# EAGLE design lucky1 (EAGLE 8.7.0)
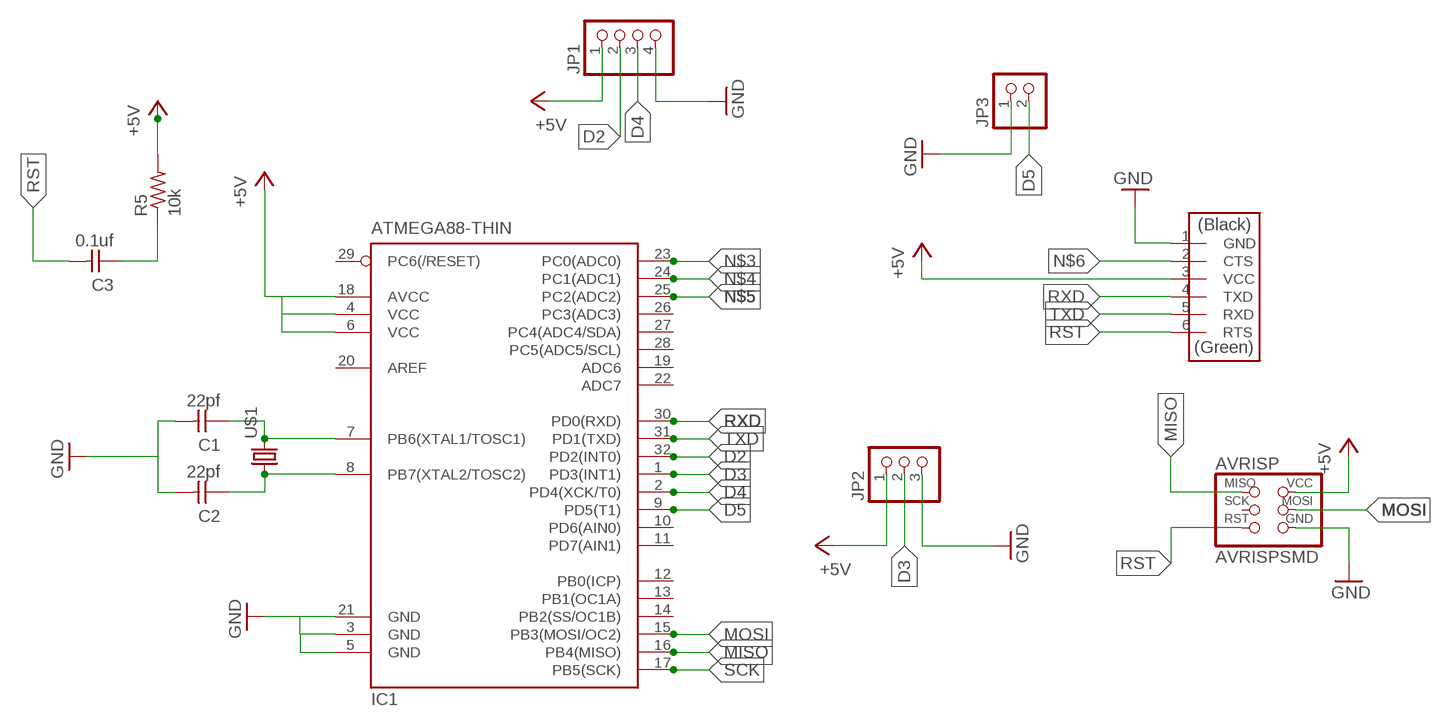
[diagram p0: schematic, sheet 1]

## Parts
AVRISP  AVRISPSMD  [2X03SMD]
C1  22pf  CAP-UNPOLARIZED  [C1206]
C2  22pf  CAP-UNPOLARIZED  [C1206]
C3  0.1uf  CAP-UNPOLARIZED  [C1206]
FTDI  FTDI-SMD-HEADER  [1X06SMD]
IC1  ATMEGA88-THIN  [TQFP32-08THIN]
JP1  PINHD-1X4  [1X04]
JP2  PINHD-1X3  [1X03]
JP3  PINHD-1X2  [1X02]
R5  10k  RES-US1206FAB  [R1206FAB]
U$1  CRYSTALHC49UP  [HC49UP]

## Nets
+5V: AVRISP.2(VCC) FTDI.3(VCC) IC1.4(VCC) IC1.6(VCC) IC1.18(AVCC) JP1.1 JP2.1 R5.2
D2: IC1.32(PD2(INT0)) JP1.2
D3: IC1.1(PD3(INT1)) JP2.2
D4: IC1.2(PD4(XCK/T0)) JP1.3
D5: IC1.9(PD5(T1)) JP3.2
GND: AVRISP.6(GND) C1.2 C2.2 FTDI.1(GND) IC1.3(GND) IC1.5(GND) IC1.21(GND) JP1.4 JP2.3 JP3.1
MISO: AVRISP.1(MISO) IC1.16(PB4(MISO))
MOSI: AVRISP.4(MOSI) IC1.15(PB3(MOSI/OC2))
N$1: C1.1 IC1.7(PB6(XTAL1/TOSC1)) U$1.2
N$2: C2.1 IC1.8(PB7(XTAL2/TOSC2)) U$1.1
N$3: IC1.23(PC0(ADC0))
N$4: IC1.24(PC1(ADC1))
N$5: IC1.25(PC2(ADC2))
N$6: FTDI.2(CTS)
N$8: C3.1 R5.1
RST: AVRISP.5(RST) C3.2 FTDI.6(RTS)
RXD: FTDI.4(TXD) IC1.30(PD0(RXD))
SCK: IC1.17(PB5(SCK))
TXD: FTDI.5(RXD) IC1.31(PD1(TXD))
Unconnected: AVRISP.3(SCK) IC1.10(PD6(AIN0)) IC1.11(PD7(AIN1)) IC1.12(PB0(ICP)) IC1.13(PB1(OC1A)) IC1.14(PB2(SS/OC1B)) IC1.19(ADC6) IC1.20(AREF) IC1.22(ADC7) IC1.26(PC3(ADC3)) IC1.27(PC4(ADC4/SDA)) IC1.28(PC5(ADC5/SCL)) IC1.29(PC6(/RESET))

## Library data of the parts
AVRISP = fab:AVRISP
C1-C3 = fab:CAP-UNPOLARIZED
FTDI = fab:FTDI-SMD-HEADER
IC1 = fab:ATMEGA88-THIN
JP1 = pinhead:PINHD-1X4: PIN HEADER
JP2 = pinhead:PINHD-1X3: PIN HEADER
JP3 = pinhead:PINHD-1X2: PIN HEADER
R5 = fab:RES-US: Resistor (US Symbol)
U$1 = crystal:CRYSTAL: CRYSTAL; OC_FARNELL: unknown; OC_NEWARK: unknown

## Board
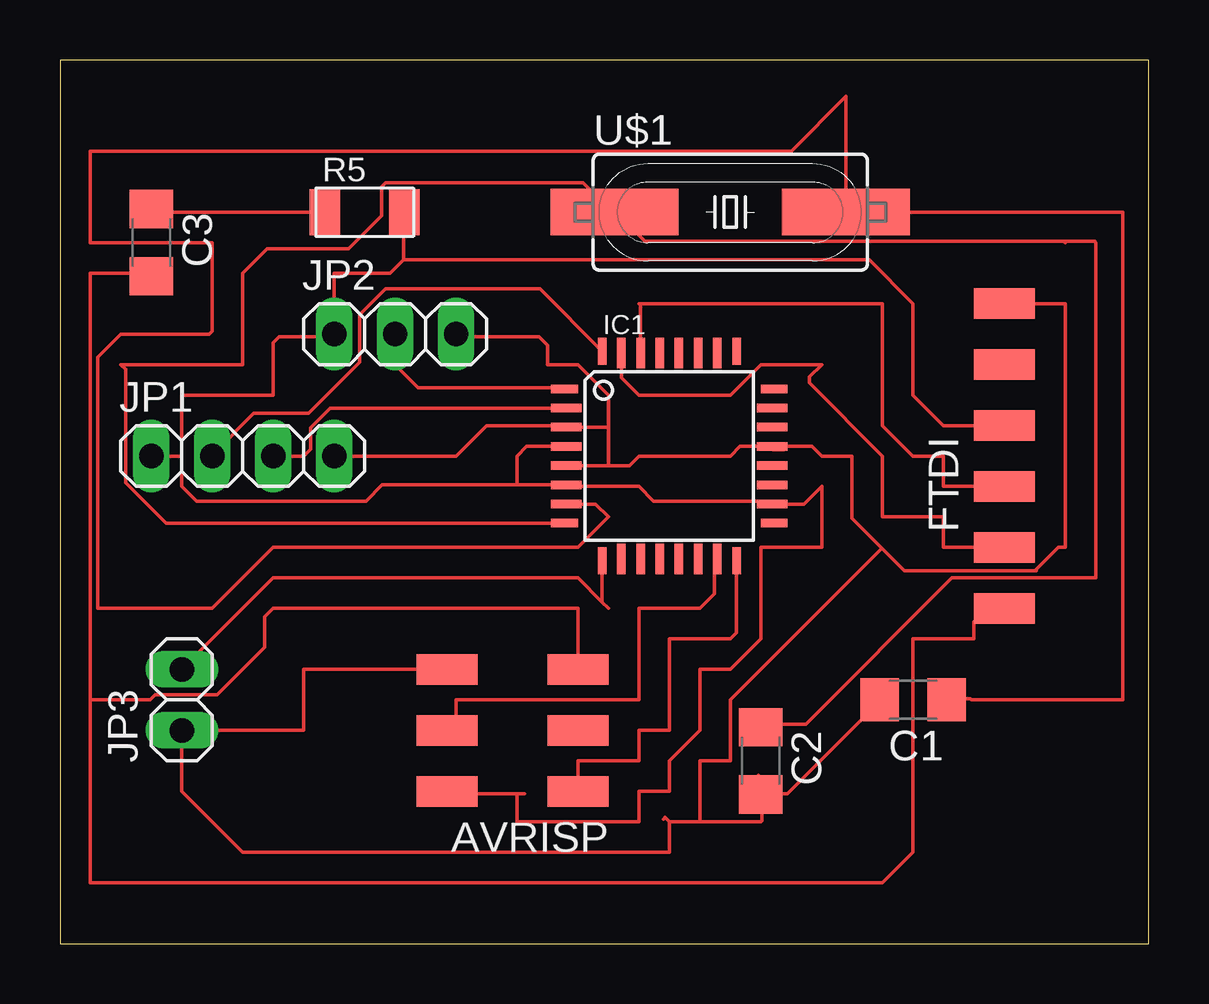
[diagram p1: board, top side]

Size 45.39 x 36.82 mm. Coordinates in mm from the lower left corner, seen from the top.
Outline: 0,0 45.39,0 45.39,36.82 0,36.82 0,0
Copper layers (1*16): Top 0.035mm / dielectric 1.5mm / Bottom 0.035mm
Design rules "default": minimum track width 6mil, minimum drill 0.35mm, track to track 6mil, track to pad 6mil, pad to pad 6mil, via to via 6mil, smd to smd 6mil, copper to edge 40mil, drill to drill 6mil, minimum pad ring 10mil, minimum via ring 8mil, stop-mask expansion 4mil, vias tented up to drill 0mil, thermal gap 10mil

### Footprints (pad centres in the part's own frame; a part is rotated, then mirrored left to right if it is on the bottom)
2X03SMD = smd 2.54 x 1.27: 1 -2.54,2.54; 2 2.92,2.54; 3 -2.54,0; 4 2.92,0; 5 -2.54,-2.54; 6 2.92,-2.54
C1206 = smd 1.6 x 1.8: 1 -1.4,0; 2 1.4,0
1X06SMD = smd 2.54 x 1.27: 1 0,6.35; 2 0,3.81; 3 0,1.27; 4 0,-1.27; 5 0,-3.81; 6 0,-6.35
TQFP32-08THIN = smd 1.118 x 0.356: 1 -4.369,2.8; 8 -4.369,-2.8; 17 4.369,-2.8; 24 4.369,2.8 | smd 1.27 x 0.356: 2 -4.293,2; 3 -4.293,1.2; 4 -4.293,0.4; 5 -4.293,-0.4; 6 -4.293,-1.2; 7 -4.293,-2; 18 4.293,-2; 19 4.293,-1.2; 20 4.293,-0.4; 21 4.293,0.4; 22 4.293,1.2; 23 4.293,2 | smd 0.356 x 1.118: 9 -2.8,-4.369; 16 2.8,-4.369; 25 2.8,4.369; 32 -2.8,4.369 | smd 0.356 x 1.27: 10 -2,-4.293; 14 1.2,-4.293; 15 2,-4.293; 26 2,4.293; 27 1.2,4.293; 31 -2,4.293 | smd 0.35 x 1.27: 11 -1.2,-4.293; 12 -0.4,-4.293; 13 0.4,-4.293; 28 0.4,4.293; 29 -0.4,4.293; 30 -1.2,4.293
1X04 = drill 1.016 long: 1 -3.81,0; 2 -1.27,0; 3 1.27,0; 4 3.81,0
1X03 = drill 1.016 long: 1 -2.54,0; 2 0,0; 3 2.54,0
1X02 = drill 1.016 long: 1 -1.27,0; 2 1.27,0
R1206FAB = smd 1.27 x 1.905: 1 -1.651,0; 2 1.651,0
HC49UP = smd 5.334 x 1.93: 1 -4.826,0; 2 4.826,0

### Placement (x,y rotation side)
AVRISP  19.05,8.89 180 top
C1  35.56,10.16 180 top
C2  29.21,7.62 270 top
C3  3.81,29.21 270 top
FTDI  39.37,20.32 0 top
IC1  25.4,20.32 0 top
JP1  7.62,20.32 0 top
JP2  13.97,25.4 0 top
JP3  5.08,10.16 90 top
R5  12.7,30.48 0 top
U$1  27.94,30.48 0 top

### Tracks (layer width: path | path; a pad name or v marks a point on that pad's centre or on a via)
+5V
  Top 0.152: 20.57,19.2 21.03,19.2 IC1.6 | IC1.6 21.18,19.05 24.13,19.05 24.74,18.44 29.57,18.44 IC1.18 31.02,18.32 31.75,19.05 31.75,16.51 29.21,16.51 29.21,12.7 27.94,11.43 26.67,11.43 26.67,8.89 25.4,7.62 25.4,6.35 24.13,6.35 24.13,5.08 19.05,5.08 19.05,6.25 | 19.36,6.25 19.05,6.25 | 19.05,6.25 16.15,6.25 AVRISP.2 | 14.33,28.5 14.33,30.48 R5.2 | JP2.1 11.43,25.6 | 39.32,21.64 FTDI.3 36.83,21.59 35.56,22.86 35.56,26.67 33.73,28.5 14.33,28.5 | 4.27,20.42 3.96,20.42 | 3.96,20.42 3.81,20.42 JP1.1 | JP2.1 11.43,25.3 9.14,25.3 8.89,25.04 8.89,22.86 5.08,22.86 5.08,20.32 | 3.96,20.42 JP1.1 | JP1.1 5.08,20.32 | 5.08,20.32 5.08,19.05 5.69,18.44 12.75,18.44 13.43,19.12 19.05,19.12 | 14.33,28.5 13.77,27.94 11.43,27.94 JP2.1 | 19.05,19.12 IC1.6 | 19.05,19.12 19.05,20.32 19.45,20.72 IC1.4
D2
  Top 0.152: JP1.2 6.4,20.42 8.08,22.1 10.36,22.1 12.5,24.23 12.5,26.21 13.56,27.28 17.78,27.28 18.44,27.28 20.01,27.28 IC1.32
D3
  Top 0.152: IC1.1 21.03,23.16 16.51,23.16 16.15,23.16 14.94,23.16 13.97,24.13 13.97,25.35 | JP2.2 13.97,25.35 | 13.97,25.35 14.02,25.3
D4
  Top 0.152: IC1.2 11.27,22.32 10.44,21.49 10.44,20.6 10.16,20.32 JP1.3
D5
  Top 0.152: 22.55,15.85 IC1.9 22.6,14.23 | 5.18,11.43 JP3.2 8.89,15.24 21.59,15.24 22.6,14.23 | 22.6,14.23 22.86,13.97
GND
  Top 0.152: 5.64,8.99 5.18,8.99 JP3.1 | 29.26,6.25 30.33,6.25 34.14,10.06 C1.2 | 29.26,6.25 C2.2 29.11,6.25 29.11,7.01 | 21.49,19.96 21.18,19.96 IC1.5 22.86,19.92 | 21.18,21.49 IC1.3 | 29.57,20.73 IC1.21 | 39.47,26.36 39.47,26.67 FTDI.1 41.91,26.67 41.91,16.51 41.6,16.51 40.64,15.54 | 40.64,15.54 35.2,15.54 34.27,16.48 | 40.64,15.54 40.69,15.54 | 30.18,20.57 29.72,20.57 IC1.21 | 11.43,20.42 JP1.4 16.51,20.32 17.78,21.59 20.93,21.59 21.03,21.49 IC1.3 | JP2.3 16.61,25.3 19.96,25.3 20.32,24.94 20.32,24.13 21.59,24.13 22.86,22.86 22.86,21.59 | 25.15,5.18 25.22,5.26 25.4,5.08 | IC1.21 28.34,20.72 27.94,20.32 24.13,20.32 23.73,19.92 22.86,19.92 | IC1.3 22.79,21.52 22.86,21.59 | 22.86,21.59 22.86,19.92 | 25.4,5.08 25.4,3.81 7.62,3.81 5.08,6.35 JP3.1 | 34.27,16.48 33.02,17.73 33.02,20.32 31.75,20.32 31.35,20.72 IC1.21 | 29.26,6.25 29.26,5.13 29.21,5.08 26.67,5.08 | 26.67,5.08 25.4,5.08 | 34.27,16.48 27.94,10.16 27.94,7.62 26.67,7.62 26.67,5.08 | JP3.1 10.16,8.89 10.16,11.43 AVRISP.6
MISO
  Top 0.152: IC1.16 28.19,15.85 28.19,12.95 27.94,12.7 25.4,12.7 25.4,8.89 24.13,8.89 24.13,7.62 21.59,7.62 AVRISP.1
MOSI
  Top 0.152: IC1.15 27.28,16 27.28,15.24 27.28,14.78 27.28,14.58 26.67,13.97 24.13,13.97 24.13,10.16 16.51,10.16 16.51,9.27 AVRISP.4 16.15,8.99
N$1
  Top 0.152: 21.18,18.29 IC1.7 22.32,18.32 22.86,17.78 21.59,16.51 8.89,16.51 6.35,13.97 1.57,13.97 1.57,24.43 2.54,25.4 6.22,25.4 6.35,25.53 6.35,29.21 1.27,29.21 1.27,33.02 30.48,33.02 32.77,35.31 U$1.2 44.3,30.48 44.3,10.16 38,10.16 37.95,10.21 37.03,10.21 C1.1
N$2
  Top 0.152: IC1.8 4.42,17.53 2.74,19.2 2.74,23.93 2.54,24.13 7.62,24.13 7.62,27.94 8.64,28.96 12.04,28.96 13.41,30.33 13.41,31.55 13.56,31.7 21.79,31.7 23.01,30.48 U$1.1 23.16,30.48 24.38,29.26 41.86,29.26 | C2.1 29.26,9.14 31.09,9.14 37.19,15.24 43.18,15.24 43.18,29.21 43.13,29.26 41.86,29.26 | 41.86,29.26 41.91,29.21
N$8
  Top 0.152: R5.1 3.81,30.48 C3.1
RST
  Top 0.152: 21.49,11.43 AVRISP.5 21.59,13.97 8.89,13.97 8.53,13.61 8.53,12.34 6.55,10.36 3.96,10.36 3.76,10.16 1.27,10.16 | FTDI.6 39.32,13.87 38.56,13.87 38.1,13.41 38.1,12.7 35.56,12.7 35.56,3.81 34.29,2.54 1.27,2.54 1.27,10.16 | C3.2 3.68,27.94 1.27,27.94 1.27,10.16
RXD
  Top 0.152: 24.23,24.99 24.23,24.69 IC1.30 24.2,26.6 24.13,26.67 34.29,26.67 34.29,21.59 35.56,20.32 36.83,20.32 36.83,19.05 FTDI.4
TXD
  Top 0.152: 23.47,24.08 23.47,24.54 IC1.31 23.4,23.59 24.13,22.86 27.94,22.86 29.21,24.13 31.75,24.13 31.24,23.62 31.24,23.37 34.29,20.32 34.29,17.78 36.83,17.78 36.83,16.51 FTDI.5 39.32,16.61 38.25,16.61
